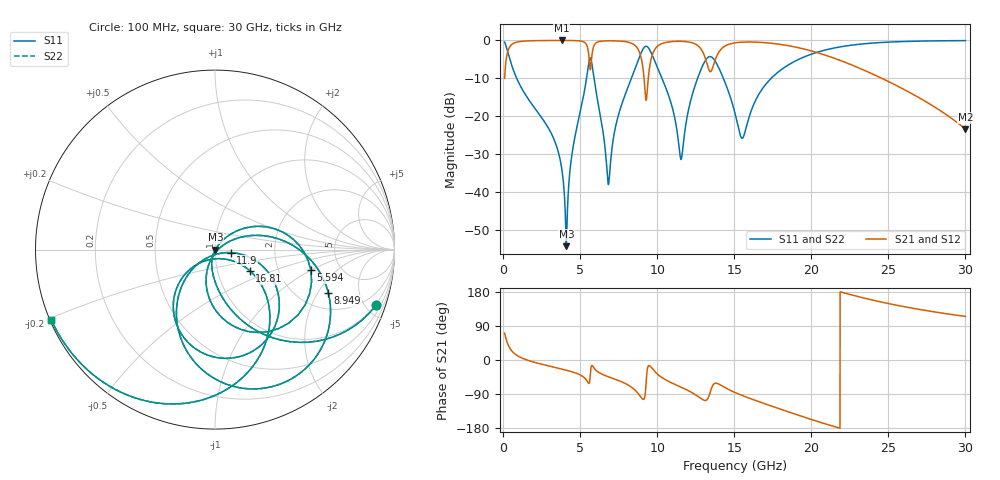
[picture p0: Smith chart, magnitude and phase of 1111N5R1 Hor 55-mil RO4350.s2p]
# GHz S MA R 50
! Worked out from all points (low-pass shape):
!   3201 points, 100 MHz to 30 GHz, reference 50 ohm
!   highest |S21| = -0.02 dB at 3.819 GHz (marker M1); lowest = -23.4 dB at 30 GHz (marker M2)
!   |S21| within 3 dB of the highest: 299.2 MHz to 5.536 GHz (5.237 GHz wide, 179 % of centre); 14.01 GHz to 20.22 GHz (6.203 GHz wide, 36.2 % of centre)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
!   lowest |S11| = -54.2 dB at 4.108 GHz (marker M3), VSWR 1.00, Z = 50.2 - j0.0716 ohm
!   |S11| at or under -10 dB: 885 MHz to 5.415 GHz (4.53 GHz wide, 144 % of centre); 5.899 GHz to 8.328 GHz (2.429 GHz wide, 34.1 % of centre); 14.3 GHz to 17.4 GHz (3.098 GHz wide, 19.6 % of centre)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
!   |S22| runs from -54.2 to -0.1 dB; largest |S21 - S12| = 0
!   S11 on the Smith chart (normalised r, x): 100 MHz: 0.93, -5.80; 5.594 GHz: 3.04, -1.00; 8.949 GHz: 2.80, -2.48; 11.9 GHz: 1.19, -0.04; 16.81 GHz: 1.43, -0.36; 30 GHz: 0.00, -0.21
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0.1  0.9486 -19.1  0.3162 70.9  0.3162 70.9  0.9486 -19.1
0.9129063  0.3072 -78.1  0.951 11.8  0.951 11.8  0.3072 -78.1
3.818812  0.0197 -109.7  0.9979 -24.1  0.9979 -24.1  0.0197 -109.7
4.108469  0.001949 -21.5  0.9976 -27.1  0.9976 -27.1  0.001949 -21.5
5.089563  0.1371 43.0  0.9761 -41.2  0.9761 -41.2  0.1371 43.0
5.594125  0.5464 -12.2  0.5494 -60.6  0.5494 -60.6  0.5464 -12.2
5.986562  0.2423 -99.9  0.907 -25.4  0.907 -25.4  0.2423 -99.9
6.846188  0.01274 -34.0  0.9867 -44.4  0.9867 -44.4  0.01274 -34.0
7.472219  0.1015 29.2  0.9818 -53.8  0.9818 -53.8  0.1015 29.2
8.948531  0.6756 -20.9  0.6014 -98.1  0.6014 -98.1  0.6756 -20.9
9.29425  0.8364 -60.0  0.1635 -53.3  0.1635 -53.3  0.8364 -60.0
10.06978  0.4141 -121.3  0.8542 -39.1  0.8542 -39.1  0.4141 -121.3
11.51806  0.02785 -88.6  0.9722 -71.1  0.9722 -71.1  0.02785 -88.6
11.90116  0.08824 -11.1  0.9613 -78.4  0.9613 -78.4  0.08824 -11.1
13.39616  0.6111 -76.0  0.3958 -91.1  0.3958 -91.1  0.6111 -76.0
13.98481  0.4396 -120.9  0.6915 -63.3  0.6915 -63.3  0.4396 -120.9
15.05  0.1095 -138.2  0.9278 -85.8  0.9278 -85.8  0.1095 -138.2
15.55456  0.05184 -77.7  0.9485 -94.2  0.9485 -94.2  0.05184 -77.7
16.80663  0.2274 -31.3  0.9393 -112.9  0.9393 -112.9  0.2274 -31.3
20.03956  0.6623 -69.5  0.7233 -157.4  0.7233 -157.4  0.6623 -69.5
25.01978  0.9494 -122.4  0.2862 148.8  0.2862 148.8  0.9494 -122.4
30  0.9927 -156.7  0.06784 115.0  0.06784 115.0  0.9927 -156.7
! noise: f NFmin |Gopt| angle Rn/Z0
0.1  0.001131  0.8451  3.292  0.001549
3.417  0.008991  0.4464  23.47  0.002609
6.743  0.04003  0.7162  43.66  0.02411
10.06  0.1067  0.8351  63.78  0.09884
13.39  0.5631  0.9567  81.86  1.676
16.7  0.09906  0.7329  98.7  0.03242
20.03  0.1042  0.7102  112.7  0.02316
23.35  0.1439  0.7669  126.6  0.02711
26.67  0.2451  0.8556  142  0.0405
30  0.589  0.939  158.2  0.07931
